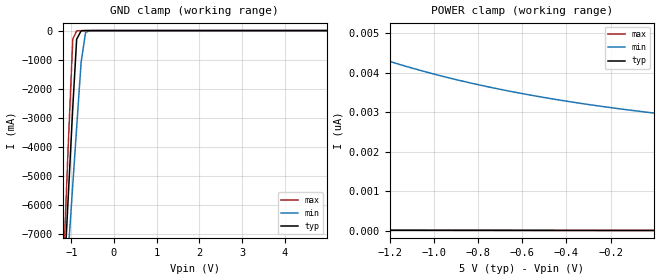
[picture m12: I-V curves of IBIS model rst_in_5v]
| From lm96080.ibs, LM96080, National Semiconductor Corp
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[Model] rst_in_5v
Model_type Input
Vinh = 2.0V
Vinl = 0.8V
C_comp   0.66pF   0.63pF   0.74pF
[Voltage Range]   5.0V   4.5V   5.5V
[Temperature Range]   25.0   125.0   -40.0
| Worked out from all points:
|   GND clamp passes 1 mA (typ) near -0.67 V on its own axis
[GND Clamp]
-5V       -119.5A    -93.09A    -149.1A
-1.175V   -8.745A    -9.913A    -7.786A
-1.07V    -5.678A    -7.603A    -3.886A
-965mV    -2.637A    -5.304A    -291.2mA
-875mV    -300.7mA   -3.351A    -8.226mA
-770mV    -8.234mA   -1.092A    -970.2uA
-665mV    -623.3uA   -60.71mA   -74.48uA
-560mV    -47.09uA   -3.609mA   -2.694uA
-470mV    -3.908uA   -378.8uA   -96.34nA
4.99V     16.91pA    0A         14.97pA
[POWER Clamp]
-5V       90.71pA    42.69nA    31.54pA
-3.575V   47.98pA    16.92nA    27.24pA
-1.61V    24.89pA    5.139nA    21.33pA
-1.565V   24.59pA    5.029nA    21.2pA
-1.415V   23.65pA    4.693nA    20.75pA
-1.205V   22.44pA    4.29nA     20.12pA
-1.055V   21.63pA    4.044nA    19.67pA
-860mV    20.65pA    3.77nA     19.08pA
-650mV    19.66pA    3.522nA    18.45pA
-455mV    18.8pA     3.327nA    17.87pA
-245mV    17.93pA    3.15nA     17.24pA
-5mV      16.97pA    2.978nA    16.52pA
